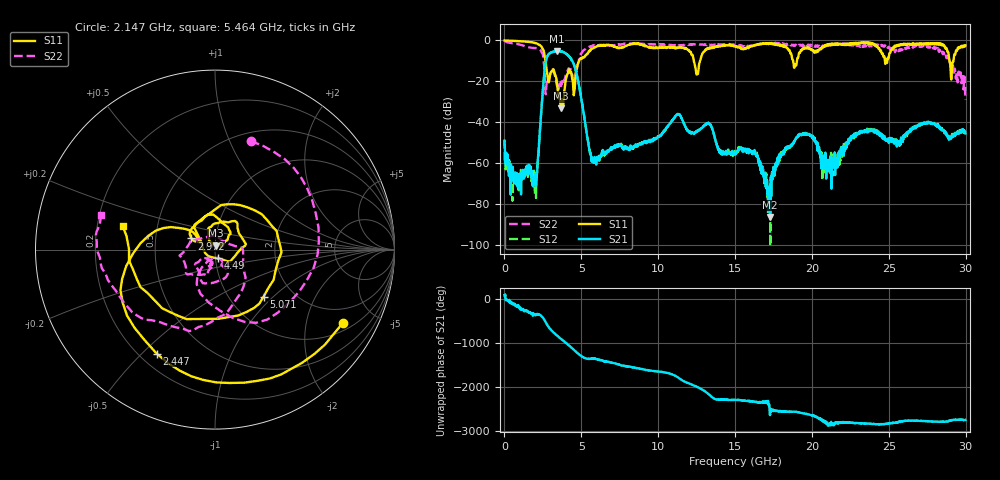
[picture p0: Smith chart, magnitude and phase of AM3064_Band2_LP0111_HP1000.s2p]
# Hz S DB R 50.0
!freq dBS11 angS11 dBS21 angS21 dBS12 angS12 dBS22 angS22
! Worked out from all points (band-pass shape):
!   1600 points, 10 MHz to 29.98 GHz, reference 50 ohm
!   highest |S21| = -5.09 dB at 3.403 GHz (marker M1); lowest = -86.2 dB at 17.27 GHz (marker M2)
!   |S21| within 3 dB of the highest: 2.776 GHz to 4.223 GHz (1.447 GHz wide, 41.4 % of centre)
!   lowest |S11| = -33.1 dB at 3.665 GHz (marker M3), VSWR 1.05, Z = 50.5 + j2.17 ohm
!   |S11| at or under -10 dB: 2.669 GHz to 4.851 GHz (2.182 GHz wide, 58 % of centre); 12.32 GHz to 12.72 GHz (403.8 MHz wide, 3.23 % of centre); 28.95 GHz to 29.2 GHz (256.8 MHz wide, 0.883 % of centre)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
!   |S22| runs from -29.0 to -0.2 dB; largest |S21 - S12| = 0.013
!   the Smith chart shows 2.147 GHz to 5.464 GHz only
!   S11 on the Smith chart (normalised r, x): 2.147 GHz: 1.31, -3.29; 2.447 GHz: 0.27, -0.55; 2.972 GHz: 0.76, +0.10; 4.49 GHz: 1.03, -0.10; 5.071 GHz: 1.43, -0.87; 5.464 GHz: 0.31, +0.11
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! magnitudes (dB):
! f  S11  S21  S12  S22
! 10 MHz  0.0  -49.4  -48.3  -0.2
! 853.5 MHz  -0.3  -71.5  -69.2  -1.8
! 2.147 GHz  -1.7  -60.3  -61.6  -3.9
! 2.447 GHz  -3.6  -29.3  -29.2  -6.1
! 2.972 GHz  -16.7  -6.1  -6.1  -16.5
! 3.403 GHz  -20.2  -5.1  -5.2  -21.8
! 3.665 GHz  -33.1  -5.4  -5.3  -23.1
! 4.49 GHz  -25.8  -11.2  -11.2  -21.7
! 5.015 GHz  -9.0  -29.2  -29.0  -6.3
! 5.071 GHz  -8.5  -31.9  -31.7  -5.5
! 5.464 GHz  -5.5  -50.6  -50.1  -3.6
! 10 GHz  -3.6  -46.7  -46.9  -1.9
! 11.31 GHz  -3.3  -36.2  -36.1  -2.7
! 12.51 GHz  -16.6  -44.4  -44.5  -1.9
! 15 GHz  -2.7  -54.6  -55.0  -2.0
! 17.27 GHz  -1.5  -86.2  -73.1  -1.4
! 18.08 GHz  -2.3  -55.8  -54.9  -1.6
! 19.99 GHz  -4.5  -47.0  -46.4  -2.2
! 21.08 GHz  -2.5  -58.3  -61.3  -2.2
! 25 GHz  -8.4  -50.1  -49.6  -3.1
! 28.31 GHz  -1.9  -42.3  -42.2  -4.6
! 29.98 GHz  -2.4  -45.4  -44.3  -29.0
